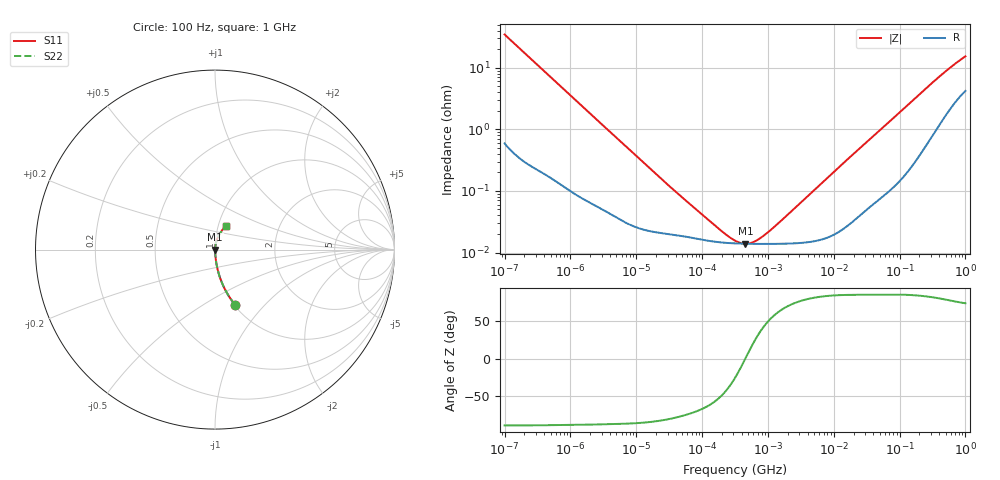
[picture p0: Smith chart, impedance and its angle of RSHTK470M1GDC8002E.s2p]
! RSHTK470M1GDC8002E  S-PARAMETER MODEL  (General Type)
! Model Generated by ELNA Corporation (http://www.ty-top.com)
! Version 1.0
! ELNA Control No.240315
! Copyright (c) 2024 ELNA CO.,LTD. All Rights Reserved.
! Products Name : CONDUCTIVE POLYMER HYBRID ALUMINUM ELECTROLYTIC CAPACITORS
! Characteristics :
!  Capacitance  :  47uF  ,  Rated voltage  :  35V
!  Operating Temp. Range  :  -55 to +125 degC  ,  Endurance  :  4000hr at 125 degC
!  Dimension D  :  6.3mm  ,  Dimension L  :  5.8mm
! Frequency Range : 100Hz - 1GHz
! External Node Assignments :
!  1  o---| |---o  2
# MHz S RI R 50
!Freq[MHz].  S11 Real  S11 Imag  S21 Real  S21 Imag  S12 Real  S12 Imag  S22 Real  S22 Imag
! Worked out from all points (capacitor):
!   401 points, 100 Hz to 1 GHz, reference 50 ohm
!   read as one part in series: C = 45.9 uF near 108 Hz
!   lowest |Z| = 13.9 mohm at 454.5 kHz (marker M1)
!   series resonance near 452.9 kHz, so ESL is about 2.7 nH
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0.0001  0.1114 -0.3063  0.8886 0.3063  0.8886 0.3063  0.1114 -0.3063
0.000113  0.0901 -0.2782  0.9099 0.2782  0.9099 0.2782  0.0901 -0.2782
0.000169  0.0436 -0.196  0.9564 0.196  0.9564 0.196  0.0436 -0.196
0.000335  0.0128 -0.1026  0.9872 0.1026  0.9872 0.1026  0.0128 -0.1026
0.000638  0.00439 -0.0548  0.9956 0.0548  0.9956 0.0548  0.00439 -0.0548
0.001488  0.00133 -0.0239  0.9987 0.0239  0.9987 0.0239  0.00133 -0.0239
0.022131  0.000212 -0.00168  0.9998 0.00168  0.9998 0.00168  0.000212 -0.00168
0.172783  0.000148 -0.000203  0.9999 0.000203  0.9999 0.000203  0.000148 -0.000203
0.248313  0.000143 -0.000117  0.9999 0.000117  0.9999 0.000117  0.000143 -0.000117
0.316228  0.000141 -6.74e-05  0.9999 6.74e-05  0.9999 6.74e-05  0.000141 -6.74e-05
0.386812  0.00014 -2.92e-05  0.9999 2.92e-05  0.9999 2.92e-05  0.00014 -2.92e-05
0.454465  0.000139 6.3e-07  0.9999 -6.3e-07  0.9999 -6.3e-07  0.000139 6.3e-07
0.533949  0.000138 3.05e-05  0.9999 -3.05e-05  0.9999 -3.05e-05  0.000138 3.05e-05
0.627336  0.000138 6.12e-05  0.9999 -6.12e-05  0.9999 -6.12e-05  0.000138 6.12e-05
0.901571  0.000138 0.000137  0.9999 -0.000137  0.9999 -0.000137  0.000138 0.000137
1.522299  0.000139 0.000283  0.9999 -0.000283  0.9999 -0.000283  0.000139 0.000283
4.704354  0.000151 0.00095  0.9998 -0.00095  0.9998 -0.00095  0.000151 0.00095
69.9842  0.00117 0.0132  0.9988 -0.0132  0.9988 -0.0132  0.00117 0.0132
176.8072  0.00412 0.0324  0.9959 -0.0324  0.9959 -0.0324  0.00412 0.0324
395.8221  0.016 0.068  0.984 -0.068  0.984 -0.068  0.016 0.068
668.3439  0.0359 0.1024  0.9641 -0.1024  0.9641 -0.1024  0.0359 0.1024
1000  0.0592 0.1332  0.9408 -0.1332  0.9408 -0.1332  0.0592 0.1332
